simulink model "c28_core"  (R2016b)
settings: Solver=FixedStepDiscrete  StartTime=0.0  StopTime=inf  RelTol=1e-3  EnableMultiTasking=on
undefined symbols (not defined in the file or in its folder): A, ADCIN0, ADCIN1, ADCINA0, ADCINB0, bit, Compare, conversion, DCAEVT1, DCAEVT1FILT, Digital, Down, ended, Event, Filtered, GPTRIP1SEL, GPTRIP2SEL, input, Module, of, Single, start, Trip, TZ1, TZ2, Up, version, Zone
libraries: c2802xlib x36, c280xlib x4, f28M35x_C28x_lib x1, c2000lib x1

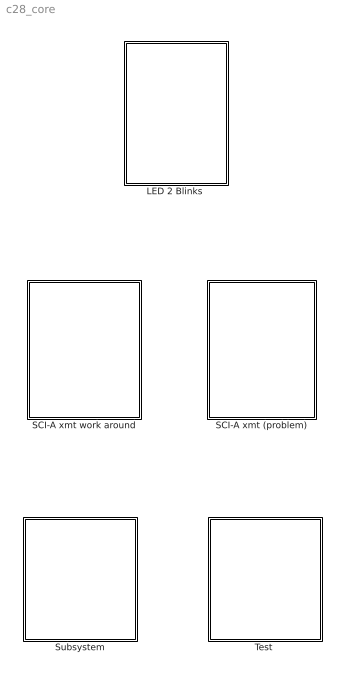
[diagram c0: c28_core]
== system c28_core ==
  "LED 2 Blinks " : Subsystem
  SCI-A xmt (problem) : Subsystem  Commented=on
  SCI-A xmt work around : Subsystem
  Subsystem : Subsystem  Commented=on
  "Test " : Subsystem

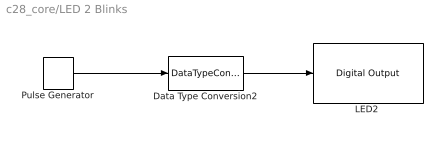
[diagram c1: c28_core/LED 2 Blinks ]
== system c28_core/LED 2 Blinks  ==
  Data Type Conversion2 : DataTypeConversion  OutDataTypeStr=boolean
  "LED2 " : f28M35x_C28x_lib/Digital Output  GPIO_Number=GPIO68~GPIO71  GPIO_Bit0=off  GPIO_BIT0_Toggle=off  GPIO_Bit1=off  GPIO_BIT1_Toggle=off  GPIO_Bit2=off  GPIO_BIT2_Toggle=off  GPIO_Bit3=off  GPIO_BIT3_Toggle=off  GPIO_Bit4=off  GPIO_BIT4_Toggle=off  GPIO_Bit5=off  GPIO_BIT5_Toggle=off  GPIO_Bit6=on  GPIO_BIT6_Toggle=off  GPIO_Bit7=off  GPIO_BIT7_Toggle=off
  Pulse Generator : DiscretePulseGenerator  PulseType=Time based  Period=1  PulseWidth=50
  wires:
  Pulse Generator/1 -> Data Type Conversion2/1
  Data Type Conversion2/1 -> "LED2 "/1

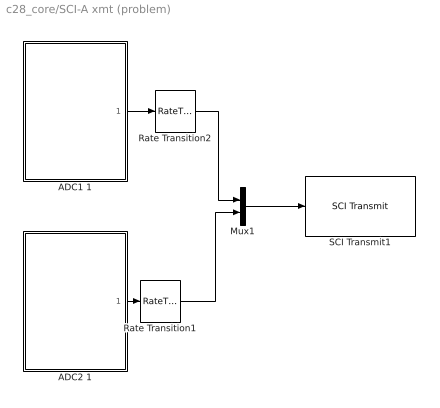
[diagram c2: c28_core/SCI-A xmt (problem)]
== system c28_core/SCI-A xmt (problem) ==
  ADC1 1 : Subsystem
  ADC2 1 : Subsystem
  Mux1 : Mux  Inputs=2
  Rate Transition1 : RateTransition  Deterministic=off
  Rate Transition2 : RateTransition  Deterministic=off
  SCI Transmit1 : c280xlib/SCI Transmit  sciModule=A  dataHead='S'  dataTail='E'  postInterrupt=off  numFifo=1
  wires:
  Mux1/1 -> SCI Transmit1/1
  ADC2 1/1(Out1) -> Rate Transition1/1
  ADC1 1/1(Out1) -> Rate Transition2/1
  Rate Transition2/1 -> Mux1/1
  Rate Transition1/1 -> Mux1/2

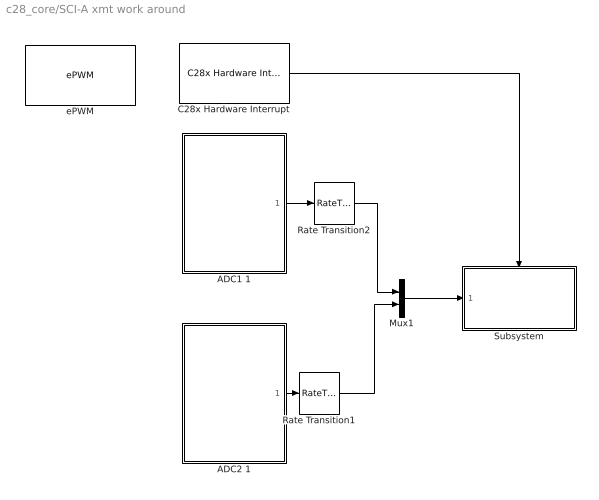
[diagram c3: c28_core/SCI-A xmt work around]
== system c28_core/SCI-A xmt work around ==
  ADC1 1 : Subsystem
  ADC2 1 : Subsystem
  C28x Hardware Interrupt : c2000lib/Scheduling/C28x Hardware Interrupt  irqnumbers=[1]  pienumbers=[1]  irqpriorities=[30]  irqpreempts=[0]  showinput=off  dspchiptype=C280X
  Mux1 : Mux  Inputs=2
  Rate Transition1 : RateTransition  Deterministic=off
  Rate Transition2 : RateTransition  Deterministic=off
  Subsystem : Subsystem
  ePWM : c2802xlib/ePWM  useModule=ePWM6  ePWMxLINKTBPRD=Not Linked  periodUnits=Seconds  timerSource=Specify via dialog  timerPeriod_clk=64000  timerPeriod_sec=0.0001  tbshadow=Counter equals to zero  countingMode=Up-Down  phaseActiveEnable=Disable  phaseDirection=Count down after sync  phaseActive=0  synchronizationEnable=off  dcaevt1Sync=off  dcbevt1Sync=off  synchronizationOption=Disable  clockPrescale=1  HSclockPrescale=1  enswap=off  ePWMxAStatus=on  ePWMxAactionLogic1=Set  ePWMxAactionLogic2=Clear  ePWMxAactionLogic3=Clear  ePWMxAactionLogic4=Set  ePWMxAactionLogic5=Do nothing  ePWMxAactionLogic6=Do nothing  ePWMxALoadMode=Load on counter equals to zero (CTR=Zero)  ePWMxACSFenable=off  ePWMxACSFvalue=Forcing disable  ePWMxASFreload=Zero  ePWMxBStatus=on  ePWMxBactionLogic1=Set  ePWMxBactionLogic2=Clear  ePWMxBactionLogic3=Do nothing  ePWMxBactionLogic4=Do nothing  ePWMxBactionLogic5=Clear  ePWMxBactionLogic6=Set  ePWMxBLoadMode=Load on counter equals to zero (CTR=Zero)  ePWMxBCSFenable=off  ePWMxBCSFvalue=Forcing disable  ePWMxBSFreload=Zero  ePWNxBOutWay=off  ePWMxLINKCMPA=Not Linked  CMPAUnits=Clock cycles  CMPASource=Specify via dialog  CMPAValue_per=50  CMPAValue_clk=32000  enCMPAshadow=Counter equals to zero  ePWMxLINKCMPB=Not Linked  CMPBUnits=Clock cycles  CMPBSource=Specify via dialog  CMPBValue_per=50  CMPBValue_clk=32000  enCMPBshadow=Counter equals to zero  ePWMxLINKCMPC=Not Linked  CMPCUnits=Clock cycles  CMPCSource=Specify via dialog  CMPCValue_per=50  CMPCValue_clk=32000  enCMPCshadow=Counter equals to zero  ePWMxLINKCMPD=Not Linked  CMPDUnits=Clock cycles  CMPDSource=Specify via dialog  CMPDValue_per=50  CMPDValue_clk=32000  enCMPDshadow=Counter equals to zero  enableDBePWMxA=off  enableDBePWMxB=off  enhalfcycle=off  DBpolarity=Active high (AH)  DBedgeDelay=Positive  DBSource_ePWMxA=ePWMxA  DBSource_ePWMxB=ePWMxA  DBperiodSource=Specify via dialog  REDperiod=0  FEDperiod=0  adcstartModuleA=off  adcrequestEventA=First event  adcstartEventA=Digital Compare Module A Event 1 start of conversion (DCAEVT1.soc)  adcstartEventA_type2=Digital Compare Module A Event 1 start of conversion (DCAEVT1.soc)  adcstartModuleB=off  adcrequestEventB=First event  adcstartEventB=Counter equals to zero (CTR=Zero)  adcstartEventB_type2=Counter equals to zero (CTR=Zero)  intEn=on  intPrd=First event  intSel=Counter equals to zero (CTR=Zero)  intSel_type2=Counter equals to zero (CTR=Zero)  hrpe=off  enHRPWM=off  HRPWM_LoadMode=Counter equals to period (CTR=PRD)  HRPWM_CTLMode=Duty or Period control mode  HRPWM_EDGMode=Both edge  hrpeb=off  enHRPWMB=off  HRPWM_LoadModeB=Counter equals to zero (CTR=ZERO)  HRPWM_CTLModeB=Duty or Period control mode  HRPWM_EDGModeB=Both edge  enSFO=on  enautoconv=on  chopperEnable=off  chopperFrequency=1  chopperFirstwidth=1  chopperDuty=12.5%  tripZonesource=Specify via dialog  tzselOSHT1=off  tzselOSHT2=off  tzselOSHT3=off  tzselOSHDCAEV1=off  tzselOSHDCBEV1=off  tzselCBC1=off  tzselCBC2=off  tzselCBC3=off  tzselCBCDCAEV2=off  tzselCBCDCBEV2=off  tzselOSHT4=off  tzselOSHT5=off  tzselOSHT6=off  tzselCBC4=off  tzselCBC5=off  tzselCBC6=off  enTzOstIntr=off  enTzCbcIntr=off  enTzDCAEVT1Intr=off  enTzDCAEVT2Intr=off  enTzDCBEVT1Intr=off  enTzDCBEVT2Intr=off  ePWMxAforced=No action  ePWMxBforced=No action  DCAEVT1forced=No action  DCBEVT1forced=No action  DCAEVT2forced=No action  DCBEVT2forced=No action  dcah=Trip Zone 1 input (TZ1)  dcal=Trip Zone 2 input (TZ2)  dcbh=Trip Zone 1 input (TZ1)  dcbl=Trip Zone 2 input (TZ2)  dcah_type2=GPTRIP1SEL/(TZ1)  dcal_type2=GPTRIP2SEL/(TZ2)  dcbh_type2=GPTRIP1SEL/(TZ1)  dcbl_type2=GPTRIP2SEL/(TZ2)  gendcaevt1=Event disabled  gendcaevt2=Event disabled  gendcbevt1=Event disabled  gendcbevt2=Event disabled  dcaevt1src=DCAEVT1 with sync  dcaevt2src=DCAEVT2 with sync  dcbevt1src=DCBEVT1 with sync  dcbevt2src=DCBEVT2 with sync  pulsesel=Counter equals to zero (CTR=Zero)  blankinv=off  blankoffset=0  blankwidth=0  evsrcsel=Filtered version of DCAEVT1 (DCAEVT1FILT)  encape=off  PwmType=Concerto
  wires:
  Mux1/1 -> Subsystem/1(In1)
  C28x Hardware Interrupt/1 -> Subsystem/Trigger
  ADC2 1/1(Out1) -> Rate Transition1/1
  ADC1 1/1(Out1) -> Rate Transition2/1
  Rate Transition2/1 -> Mux1/1
  Rate Transition1/1 -> Mux1/2

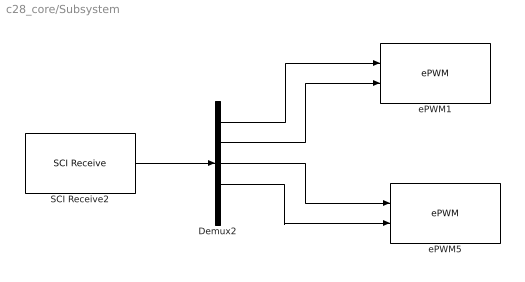
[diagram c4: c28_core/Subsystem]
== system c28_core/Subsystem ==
  Demux2 : Demux  Outputs=5
  SCI Receive2 : c280xlib/SCI Receive  sciModule=A  dataHead='S'  dataTail='E'  dataType=uint16  dataDim=5  initValue=0  errOption=Output the last received value  errValue=0  sampleTime=0.01  outputStatus=off  postInterrupt=off  numFifo=1
  ePWM1 : c2802xlib/ePWM  useModule=ePWM1  ePWMxLINKTBPRD=Not Linked  periodUnits=Clock cycles  timerSource=Specify via dialog  timerPeriod_clk=64000  timerPeriod_sec=0.0001  tbshadow=Counter equals to zero  countingMode=Up-Down  phaseActiveEnable=Disable  phaseDirection=Count down after sync  phaseActive=0  synchronizationEnable=off  dcaevt1Sync=off  dcbevt1Sync=off  synchronizationOption=Disable  clockPrescale=1  HSclockPrescale=1  enswap=off  ePWMxAStatus=on  ePWMxAactionLogic1=Set  ePWMxAactionLogic2=Clear  ePWMxAactionLogic3=Clear  ePWMxAactionLogic4=Set  ePWMxAactionLogic5=Do nothing  ePWMxAactionLogic6=Do nothing  ePWMxALoadMode=Load on counter equals to zero (CTR=Zero)  ePWMxACSFenable=off  ePWMxACSFvalue=Forcing disable  ePWMxASFreload=Zero  ePWMxBStatus=on  ePWMxBactionLogic1=Set  ePWMxBactionLogic2=Clear  ePWMxBactionLogic3=Do nothing  ePWMxBactionLogic4=Do nothing  ePWMxBactionLogic5=Clear  ePWMxBactionLogic6=Set  ePWMxBLoadMode=Load on counter equals to zero (CTR=Zero)  ePWMxBCSFenable=off  ePWMxBCSFvalue=Forcing disable  ePWMxBSFreload=Zero  ePWNxBOutWay=off  ePWMxLINKCMPA=Not Linked  CMPAUnits=Clock cycles  CMPASource=Input port  CMPAValue_per=50  CMPAValue_clk=32000  enCMPAshadow=Counter equals to zero  ePWMxLINKCMPB=Not Linked  CMPBUnits=Clock cycles  CMPBSource=Input port  CMPBValue_per=50  CMPBValue_clk=32000  enCMPBshadow=Counter equals to zero  ePWMxLINKCMPC=Not Linked  CMPCUnits=Clock cycles  CMPCSource=Specify via dialog  CMPCValue_per=50  CMPCValue_clk=32000  enCMPCshadow=Counter equals to zero  ePWMxLINKCMPD=Not Linked  CMPDUnits=Clock cycles  CMPDSource=Specify via dialog  CMPDValue_per=50  CMPDValue_clk=32000  enCMPDshadow=Counter equals to zero  enableDBePWMxA=off  enableDBePWMxB=off  enhalfcycle=off  DBpolarity=Active high (AH)  DBedgeDelay=Positive  DBSource_ePWMxA=ePWMxA  DBSource_ePWMxB=ePWMxA  DBperiodSource=Specify via dialog  REDperiod=0  FEDperiod=0  adcstartModuleA=off  adcrequestEventA=First event  adcstartEventA=Digital Compare Module A Event 1 start of conversion (DCAEVT1.soc)  adcstartEventA_type2=Digital Compare Module A Event 1 start of conversion (DCAEVT1.soc)  adcstartModuleB=off  adcrequestEventB=First event  adcstartEventB=Counter equals to zero (CTR=Zero)  adcstartEventB_type2=Counter equals to zero (CTR=Zero)  intEn=off  intPrd=First event  intSel=Counter equals to zero (CTR=Zero)  intSel_type2=Counter equals to zero (CTR=Zero)  hrpe=off  enHRPWM=off  HRPWM_LoadMode=Counter equals to period (CTR=PRD)  HRPWM_CTLMode=Duty or Period control mode  HRPWM_EDGMode=Both edge  hrpeb=off  enHRPWMB=off  HRPWM_LoadModeB=Counter equals to zero (CTR=ZERO)  HRPWM_CTLModeB=Duty or Period control mode  HRPWM_EDGModeB=Both edge  enSFO=on  enautoconv=on  chopperEnable=off  chopperFrequency=1  chopperFirstwidth=1  chopperDuty=12.5%  tripZonesource=Specify via dialog  tzselOSHT1=off  tzselOSHT2=off  tzselOSHT3=off  tzselOSHDCAEV1=off  tzselOSHDCBEV1=off  tzselCBC1=off  tzselCBC2=off  tzselCBC3=off  tzselCBCDCAEV2=off  tzselCBCDCBEV2=off  tzselOSHT4=off  tzselOSHT5=off  tzselOSHT6=off  tzselCBC4=off  tzselCBC5=off  tzselCBC6=off  enTzOstIntr=off  enTzCbcIntr=off  enTzDCAEVT1Intr=off  enTzDCAEVT2Intr=off  enTzDCBEVT1Intr=off  enTzDCBEVT2Intr=off  ePWMxAforced=No action  ePWMxBforced=No action  DCAEVT1forced=No action  DCBEVT1forced=No action  DCAEVT2forced=No action  DCBEVT2forced=No action  dcah=Trip Zone 1 input (TZ1)  dcal=Trip Zone 2 input (TZ2)  dcbh=Trip Zone 1 input (TZ1)  dcbl=Trip Zone 2 input (TZ2)  dcah_type2=GPTRIP1SEL/(TZ1)  dcal_type2=GPTRIP2SEL/(TZ2)  dcbh_type2=GPTRIP1SEL/(TZ1)  dcbl_type2=GPTRIP2SEL/(TZ2)  gendcaevt1=Event disabled  gendcaevt2=Event disabled  gendcbevt1=Event disabled  gendcbevt2=Event disabled  dcaevt1src=DCAEVT1 with sync  dcaevt2src=DCAEVT2 with sync  dcbevt1src=DCBEVT1 with sync  dcbevt2src=DCBEVT2 with sync  pulsesel=Counter equals to zero (CTR=Zero)  blankinv=off  blankoffset=0  blankwidth=0  evsrcsel=Filtered version of DCAEVT1 (DCAEVT1FILT)  encape=off  PwmType=Concerto
  ePWM5 : c2802xlib/ePWM  useModule=ePWM2  ePWMxLINKTBPRD=Not Linked  periodUnits=Clock cycles  timerSource=Specify via dialog  timerPeriod_clk=64000  timerPeriod_sec=0.0001  tbshadow=Counter equals to zero  countingMode=Up-Down  phaseActiveEnable=Disable  phaseDirection=Count down after sync  phaseActive=0  synchronizationEnable=off  dcaevt1Sync=off  dcbevt1Sync=off  synchronizationOption=Disable  clockPrescale=1  HSclockPrescale=1  enswap=off  ePWMxAStatus=on  ePWMxAactionLogic1=Set  ePWMxAactionLogic2=Clear  ePWMxAactionLogic3=Clear  ePWMxAactionLogic4=Set  ePWMxAactionLogic5=Do nothing  ePWMxAactionLogic6=Do nothing  ePWMxALoadMode=Load on counter equals to zero (CTR=Zero)  ePWMxACSFenable=off  ePWMxACSFvalue=Forcing disable  ePWMxASFreload=Zero  ePWMxBStatus=on  ePWMxBactionLogic1=Set  ePWMxBactionLogic2=Clear  ePWMxBactionLogic3=Do nothing  ePWMxBactionLogic4=Do nothing  ePWMxBactionLogic5=Clear  ePWMxBactionLogic6=Set  ePWMxBLoadMode=Load on counter equals to zero (CTR=Zero)  ePWMxBCSFenable=off  ePWMxBCSFvalue=Forcing disable  ePWMxBSFreload=Zero  ePWNxBOutWay=off  ePWMxLINKCMPA=Not Linked  CMPAUnits=Clock cycles  CMPASource=Input port  CMPAValue_per=50  CMPAValue_clk=32000  enCMPAshadow=Counter equals to zero  ePWMxLINKCMPB=Not Linked  CMPBUnits=Clock cycles  CMPBSource=Input port  CMPBValue_per=50  CMPBValue_clk=32000  enCMPBshadow=Counter equals to zero  ePWMxLINKCMPC=Not Linked  CMPCUnits=Clock cycles  CMPCSource=Specify via dialog  CMPCValue_per=50  CMPCValue_clk=32000  enCMPCshadow=Counter equals to zero  ePWMxLINKCMPD=Not Linked  CMPDUnits=Clock cycles  CMPDSource=Specify via dialog  CMPDValue_per=50  CMPDValue_clk=32000  enCMPDshadow=Counter equals to zero  enableDBePWMxA=off  enableDBePWMxB=off  enhalfcycle=off  DBpolarity=Active high (AH)  DBedgeDelay=Positive  DBSource_ePWMxA=ePWMxA  DBSource_ePWMxB=ePWMxA  DBperiodSource=Specify via dialog  REDperiod=0  FEDperiod=0  adcstartModuleA=off  adcrequestEventA=First event  adcstartEventA=Digital Compare Module A Event 1 start of conversion (DCAEVT1.soc)  adcstartEventA_type2=Digital Compare Module A Event 1 start of conversion (DCAEVT1.soc)  adcstartModuleB=off  adcrequestEventB=First event  adcstartEventB=Counter equals to zero (CTR=Zero)  adcstartEventB_type2=Counter equals to zero (CTR=Zero)  intEn=off  intPrd=First event  intSel=Counter equals to zero (CTR=Zero)  intSel_type2=Counter equals to zero (CTR=Zero)  hrpe=off  enHRPWM=off  HRPWM_LoadMode=Counter equals to period (CTR=PRD)  HRPWM_CTLMode=Duty or Period control mode  HRPWM_EDGMode=Both edge  hrpeb=off  enHRPWMB=off  HRPWM_LoadModeB=Counter equals to zero (CTR=ZERO)  HRPWM_CTLModeB=Duty or Period control mode  HRPWM_EDGModeB=Both edge  enSFO=on  enautoconv=on  chopperEnable=off  chopperFrequency=1  chopperFirstwidth=1  chopperDuty=12.5%  tripZonesource=Specify via dialog  tzselOSHT1=off  tzselOSHT2=off  tzselOSHT3=off  tzselOSHDCAEV1=off  tzselOSHDCBEV1=off  tzselCBC1=off  tzselCBC2=off  tzselCBC3=off  tzselCBCDCAEV2=off  tzselCBCDCBEV2=off  tzselOSHT4=off  tzselOSHT5=off  tzselOSHT6=off  tzselCBC4=off  tzselCBC5=off  tzselCBC6=off  enTzOstIntr=off  enTzCbcIntr=off  enTzDCAEVT1Intr=off  enTzDCAEVT2Intr=off  enTzDCBEVT1Intr=off  enTzDCBEVT2Intr=off  ePWMxAforced=No action  ePWMxBforced=No action  DCAEVT1forced=No action  DCBEVT1forced=No action  DCAEVT2forced=No action  DCBEVT2forced=No action  dcah=Trip Zone 1 input (TZ1)  dcal=Trip Zone 2 input (TZ2)  dcbh=Trip Zone 1 input (TZ1)  dcbl=Trip Zone 2 input (TZ2)  dcah_type2=GPTRIP1SEL/(TZ1)  dcal_type2=GPTRIP2SEL/(TZ2)  dcbh_type2=GPTRIP1SEL/(TZ1)  dcbl_type2=GPTRIP2SEL/(TZ2)  gendcaevt1=Event disabled  gendcaevt2=Event disabled  gendcbevt1=Event disabled  gendcbevt2=Event disabled  dcaevt1src=DCAEVT1 with sync  dcaevt2src=DCAEVT2 with sync  dcbevt1src=DCBEVT1 with sync  dcbevt2src=DCBEVT2 with sync  pulsesel=Counter equals to zero (CTR=Zero)  blankinv=off  blankoffset=0  blankwidth=0  evsrcsel=Filtered version of DCAEVT1 (DCAEVT1FILT)  encape=off  PwmType=Concerto
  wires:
  SCI Receive2/1 -> Demux2/1
  Demux2/4 -> ePWM5/2
  Demux2/3 -> ePWM5/1
  Demux2/2 -> ePWM1/2
  Demux2/1 -> ePWM1/1

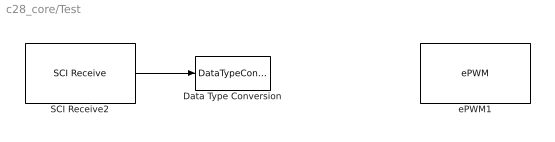
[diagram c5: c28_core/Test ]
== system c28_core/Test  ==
  Data Type Conversion : DataTypeConversion  OutDataTypeStr=uint16
  SCI Receive2 : c280xlib/SCI Receive  sciModule=A  dataHead='S'  dataTail='E'  dataType=uint8  dataDim=1  initValue=0  errOption=Output the last received value  errValue=0  sampleTime=0.01  outputStatus=off  postInterrupt=off  numFifo=1
  ePWM1 : c2802xlib/ePWM  useModule=ePWM1  ePWMxLINKTBPRD=Not Linked  periodUnits=Clock cycles  timerSource=Specify via dialog  timerPeriod_clk=64000  timerPeriod_sec=0.0001  tbshadow=Counter equals to zero  countingMode=Up-Down  phaseActiveEnable=Disable  phaseDirection=Count down after sync  phaseActive=0  synchronizationEnable=off  dcaevt1Sync=off  dcbevt1Sync=off  synchronizationOption=Disable  clockPrescale=1  HSclockPrescale=1  enswap=off  ePWMxAStatus=on  ePWMxAactionLogic1=Set  ePWMxAactionLogic2=Clear  ePWMxAactionLogic3=Clear  ePWMxAactionLogic4=Set  ePWMxAactionLogic5=Do nothing  ePWMxAactionLogic6=Do nothing  ePWMxALoadMode=Load on counter equals to zero (CTR=Zero)  ePWMxACSFenable=off  ePWMxACSFvalue=Forcing disable  ePWMxASFreload=Zero  ePWMxBStatus=on  ePWMxBactionLogic1=Set  ePWMxBactionLogic2=Clear  ePWMxBactionLogic3=Do nothing  ePWMxBactionLogic4=Do nothing  ePWMxBactionLogic5=Clear  ePWMxBactionLogic6=Set  ePWMxBLoadMode=Load on counter equals to zero (CTR=Zero)  ePWMxBCSFenable=off  ePWMxBCSFvalue=Forcing disable  ePWMxBSFreload=Zero  ePWNxBOutWay=off  ePWMxLINKCMPA=Not Linked  CMPAUnits=Clock cycles  CMPASource=Input port  CMPAValue_per=50  CMPAValue_clk=32000  enCMPAshadow=Counter equals to zero  ePWMxLINKCMPB=Not Linked  CMPBUnits=Clock cycles  CMPBSource=Specify via dialog  CMPBValue_per=50  CMPBValue_clk=32000  enCMPBshadow=Counter equals to zero  ePWMxLINKCMPC=Not Linked  CMPCUnits=Clock cycles  CMPCSource=Specify via dialog  CMPCValue_per=50  CMPCValue_clk=32000  enCMPCshadow=Counter equals to zero  ePWMxLINKCMPD=Not Linked  CMPDUnits=Clock cycles  CMPDSource=Specify via dialog  CMPDValue_per=50  CMPDValue_clk=32000  enCMPDshadow=Counter equals to zero  enableDBePWMxA=off  enableDBePWMxB=off  enhalfcycle=off  DBpolarity=Active high (AH)  DBedgeDelay=Positive  DBSource_ePWMxA=ePWMxA  DBSource_ePWMxB=ePWMxA  DBperiodSource=Specify via dialog  REDperiod=0  FEDperiod=0  adcstartModuleA=off  adcrequestEventA=First event  adcstartEventA=Digital Compare Module A Event 1 start of conversion (DCAEVT1.soc)  adcstartEventA_type2=Digital Compare Module A Event 1 start of conversion (DCAEVT1.soc)  adcstartModuleB=off  adcrequestEventB=First event  adcstartEventB=Counter equals to zero (CTR=Zero)  adcstartEventB_type2=Counter equals to zero (CTR=Zero)  intEn=off  intPrd=First event  intSel=Counter equals to zero (CTR=Zero)  intSel_type2=Counter equals to zero (CTR=Zero)  hrpe=off  enHRPWM=off  HRPWM_LoadMode=Counter equals to period (CTR=PRD)  HRPWM_CTLMode=Duty or Period control mode  HRPWM_EDGMode=Both edge  hrpeb=off  enHRPWMB=off  HRPWM_LoadModeB=Counter equals to zero (CTR=ZERO)  HRPWM_CTLModeB=Duty or Period control mode  HRPWM_EDGModeB=Both edge  enSFO=on  enautoconv=on  chopperEnable=off  chopperFrequency=1  chopperFirstwidth=1  chopperDuty=12.5%  tripZonesource=Specify via dialog  tzselOSHT1=off  tzselOSHT2=off  tzselOSHT3=off  tzselOSHDCAEV1=off  tzselOSHDCBEV1=off  tzselCBC1=off  tzselCBC2=off  tzselCBC3=off  tzselCBCDCAEV2=off  tzselCBCDCBEV2=off  tzselOSHT4=off  tzselOSHT5=off  tzselOSHT6=off  tzselCBC4=off  tzselCBC5=off  tzselCBC6=off  enTzOstIntr=off  enTzCbcIntr=off  enTzDCAEVT1Intr=off  enTzDCAEVT2Intr=off  enTzDCBEVT1Intr=off  enTzDCBEVT2Intr=off  ePWMxAforced=No action  ePWMxBforced=No action  DCAEVT1forced=No action  DCBEVT1forced=No action  DCAEVT2forced=No action  DCBEVT2forced=No action  dcah=Trip Zone 1 input (TZ1)  dcal=Trip Zone 2 input (TZ2)  dcbh=Trip Zone 1 input (TZ1)  dcbl=Trip Zone 2 input (TZ2)  dcah_type2=GPTRIP1SEL/(TZ1)  dcal_type2=GPTRIP2SEL/(TZ2)  dcbh_type2=GPTRIP1SEL/(TZ1)  dcbl_type2=GPTRIP2SEL/(TZ2)  gendcaevt1=Event disabled  gendcaevt2=Event disabled  gendcbevt1=Event disabled  gendcbevt2=Event disabled  dcaevt1src=DCAEVT1 with sync  dcaevt2src=DCAEVT2 with sync  dcbevt1src=DCBEVT1 with sync  dcbevt2src=DCBEVT2 with sync  pulsesel=Counter equals to zero (CTR=Zero)  blankinv=off  blankoffset=0  blankwidth=0  evsrcsel=Filtered version of DCAEVT1 (DCAEVT1FILT)  encape=off  PwmType=Concerto
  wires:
  SCI Receive2/1 -> Data Type Conversion/1

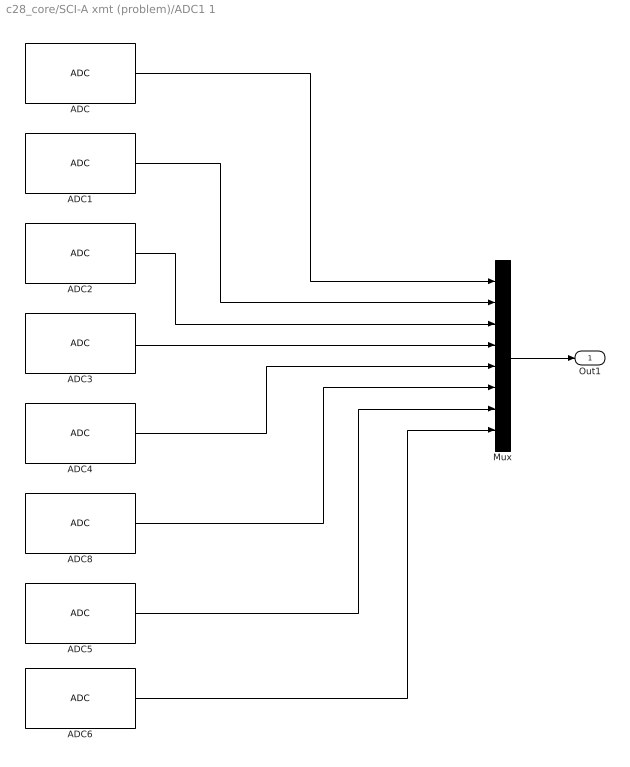
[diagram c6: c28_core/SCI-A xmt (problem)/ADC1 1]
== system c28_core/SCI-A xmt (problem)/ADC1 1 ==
  ADC : c2802xlib/ADC  ADCModule=1  samplingMode=Single sample mode  ADCResolution=12-bit (Single-ended input)  useSOC1=SOC0  useSOC2=SOC0_SOC1  SOCAcquisitionWindow=10  SOCTriggerSource=Software  SOCInterruptTrigger=No ADCINT  Ts=0.0001  dType=uint16  postInterrupt=off  interruptSel=ADCINT1  ADCINTContinuous=off  endma=off  chdma=1  blkParamProc=Concerto  conv1=ADCINA0  conv2=ADCINA0 and ADCINB0  conv1_Type4=ADCIN0  conv2_Type4=ADCIN0 and ADCIN1
  ADC1 : c2802xlib/ADC  ADCModule=1  samplingMode=Single sample mode  ADCResolution=12-bit (Single-ended input)  useSOC1=SOC1  useSOC2=SOC0_SOC1  SOCAcquisitionWindow=10  SOCTriggerSource=Software  SOCInterruptTrigger=No ADCINT  Ts=0.0001  dType=uint16  postInterrupt=off  interruptSel=ADCINT1  ADCINTContinuous=off  endma=off  chdma=1  blkParamProc=Concerto  conv1=ADCINB0  conv2=ADCINA0 and ADCINB0  conv1_Type4=ADCIN0  conv2_Type4=ADCIN0 and ADCIN1
  ADC2 : c2802xlib/ADC  ADCModule=1  samplingMode=Single sample mode  ADCResolution=12-bit (Single-ended input)  useSOC1=SOC2  useSOC2=SOC0_SOC1  SOCAcquisitionWindow=10  SOCTriggerSource=Software  SOCInterruptTrigger=No ADCINT  Ts=0.0001  dType=uint16  postInterrupt=off  interruptSel=ADCINT1  ADCINTContinuous=off  endma=off  chdma=1  blkParamProc=Concerto  conv1=ADCINA2  conv2=ADCINA0 and ADCINB0  conv1_Type4=ADCIN0  conv2_Type4=ADCIN0 and ADCIN1
  ADC3 : c2802xlib/ADC  ADCModule=1  samplingMode=Single sample mode  ADCResolution=12-bit (Single-ended input)  useSOC1=SOC3  useSOC2=SOC0_SOC1  SOCAcquisitionWindow=10  SOCTriggerSource=Software  SOCInterruptTrigger=No ADCINT  Ts=0.0001  dType=uint16  postInterrupt=off  interruptSel=ADCINT1  ADCINTContinuous=off  endma=off  chdma=1  blkParamProc=Concerto  conv1=ADCINA3  conv2=ADCINA0 and ADCINB0  conv1_Type4=ADCIN0  conv2_Type4=ADCIN0 and ADCIN1
  ADC4 : c2802xlib/ADC  ADCModule=1  samplingMode=Single sample mode  ADCResolution=12-bit (Single-ended input)  useSOC1=SOC4  useSOC2=SOC0_SOC1  SOCAcquisitionWindow=10  SOCTriggerSource=Software  SOCInterruptTrigger=No ADCINT  Ts=0.0001  dType=uint16  postInterrupt=off  interruptSel=ADCINT1  ADCINTContinuous=off  endma=off  chdma=1  blkParamProc=Concerto  conv1=ADCINA4  conv2=ADCINA0 and ADCINB0  conv1_Type4=ADCIN0  conv2_Type4=ADCIN0 and ADCIN1
  ADC5 : c2802xlib/ADC  ADCModule=1  samplingMode=Single sample mode  ADCResolution=12-bit (Single-ended input)  useSOC1=SOC6  useSOC2=SOC0_SOC1  SOCAcquisitionWindow=10  SOCTriggerSource=Software  SOCInterruptTrigger=No ADCINT  Ts=0.0001  dType=uint16  postInterrupt=off  interruptSel=ADCINT1  ADCINTContinuous=off  endma=off  chdma=1  blkParamProc=Concerto  conv1=ADCINA6  conv2=ADCINA0 and ADCINB0  conv1_Type4=ADCIN0  conv2_Type4=ADCIN0 and ADCIN1
  ADC6 : c2802xlib/ADC  ADCModule=1  samplingMode=Single sample mode  ADCResolution=12-bit (Single-ended input)  useSOC1=SOC7  useSOC2=SOC0_SOC1  SOCAcquisitionWindow=10  SOCTriggerSource=Software  SOCInterruptTrigger=No ADCINT  Ts=0.0001  dType=uint16  postInterrupt=on  interruptSel=ADCINT1  ADCINTContinuous=off  endma=off  chdma=1  blkParamProc=Concerto  conv1=ADCINA7  conv2=ADCINA0 and ADCINB0  conv1_Type4=ADCIN0  conv2_Type4=ADCIN0 and ADCIN1
  ADC8 : c2802xlib/ADC  ADCModule=1  samplingMode=Single sample mode  ADCResolution=12-bit (Single-ended input)  useSOC1=SOC5  useSOC2=SOC0_SOC1  SOCAcquisitionWindow=10  SOCTriggerSource=Software  SOCInterruptTrigger=No ADCINT  Ts=0.0001  dType=uint16  postInterrupt=off  interruptSel=ADCINT1  ADCINTContinuous=off  endma=off  chdma=1  blkParamProc=Concerto  conv1=ADCINB4  conv2=ADCINA0 and ADCINB0  conv1_Type4=ADCIN0  conv2_Type4=ADCIN0 and ADCIN1
  Mux : Mux  Inputs=8
  Out1 : Outport
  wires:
  Mux/1 -> Out1/1
  ADC/1 -> Mux/1
  ADC1/1 -> Mux/2
  ADC2/1 -> Mux/3
  ADC3/1 -> Mux/4
  ADC4/1 -> Mux/5
  ADC8/1 -> Mux/6
  ADC5/1 -> Mux/7
  ADC6/1 -> Mux/8

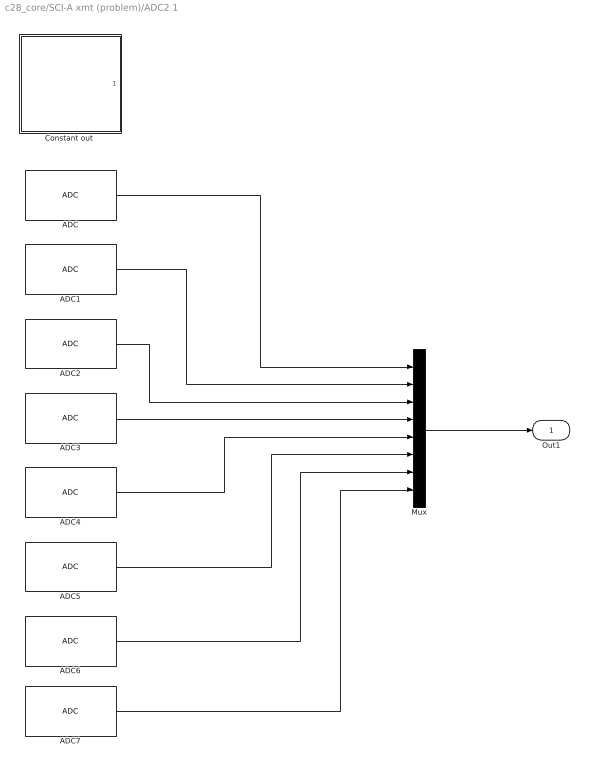
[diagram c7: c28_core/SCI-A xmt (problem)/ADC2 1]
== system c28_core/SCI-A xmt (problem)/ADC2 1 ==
  ADC : c2802xlib/ADC  ADCModule=2  samplingMode=Single sample mode  ADCResolution=12-bit (Single-ended input)  useSOC1=SOC8  useSOC2=SOC0_SOC1  SOCAcquisitionWindow=10  SOCTriggerSource=Software  SOCInterruptTrigger=No ADCINT  Ts=0.0001  dType=uint16  postInterrupt=off  interruptSel=ADCINT1  ADCINTContinuous=off  endma=off  chdma=1  blkParamProc=Concerto  conv1=ADCINA0  conv2=ADCINA0 and ADCINB0  conv1_Type4=ADCIN0  conv2_Type4=ADCIN0 and ADCIN1
  ADC1 : c2802xlib/ADC  ADCModule=2  samplingMode=Single sample mode  ADCResolution=12-bit (Single-ended input)  useSOC1=SOC9  useSOC2=SOC0_SOC1  SOCAcquisitionWindow=10  SOCTriggerSource=Software  SOCInterruptTrigger=No ADCINT  Ts=0.0001  dType=uint16  postInterrupt=off  interruptSel=ADCINT1  ADCINTContinuous=off  endma=off  chdma=1  blkParamProc=Concerto  conv1=ADCINB0  conv2=ADCINA0 and ADCINB0  conv1_Type4=ADCIN0  conv2_Type4=ADCIN0 and ADCIN1
  ADC2 : c2802xlib/ADC  ADCModule=2  samplingMode=Single sample mode  ADCResolution=12-bit (Single-ended input)  useSOC1=SOC10  useSOC2=SOC0_SOC1  SOCAcquisitionWindow=10  SOCTriggerSource=Software  SOCInterruptTrigger=No ADCINT  Ts=0.0001  dType=uint16  postInterrupt=off  interruptSel=ADCINT1  ADCINTContinuous=off  endma=off  chdma=1  blkParamProc=Concerto  conv1=ADCINA2  conv2=ADCINA0 and ADCINB0  conv1_Type4=ADCIN0  conv2_Type4=ADCIN0 and ADCIN1
  ADC3 : c2802xlib/ADC  ADCModule=2  samplingMode=Single sample mode  ADCResolution=12-bit (Single-ended input)  useSOC1=SOC11  useSOC2=SOC0_SOC1  SOCAcquisitionWindow=10  SOCTriggerSource=Software  SOCInterruptTrigger=No ADCINT  Ts=0.0001  dType=uint16  postInterrupt=off  interruptSel=ADCINT1  ADCINTContinuous=off  endma=off  chdma=1  blkParamProc=Concerto  conv1=ADCINA3  conv2=ADCINA0 and ADCINB0  conv1_Type4=ADCIN0  conv2_Type4=ADCIN0 and ADCIN1
  ADC4 : c2802xlib/ADC  ADCModule=2  samplingMode=Single sample mode  ADCResolution=12-bit (Single-ended input)  useSOC1=SOC12  useSOC2=SOC0_SOC1  SOCAcquisitionWindow=10  SOCTriggerSource=Software  SOCInterruptTrigger=No ADCINT  Ts=0.0001  dType=uint16  postInterrupt=off  interruptSel=ADCINT1  ADCINTContinuous=off  endma=off  chdma=1  blkParamProc=Concerto  conv1=ADCINA4  conv2=ADCINA0 and ADCINB0  conv1_Type4=ADCIN0  conv2_Type4=ADCIN0 and ADCIN1
  ADC5 : c2802xlib/ADC  ADCModule=2  samplingMode=Single sample mode  ADCResolution=12-bit (Single-ended input)  useSOC1=SOC13  useSOC2=SOC0_SOC1  SOCAcquisitionWindow=10  SOCTriggerSource=Software  SOCInterruptTrigger=No ADCINT  Ts=0.0001  dType=uint16  postInterrupt=off  interruptSel=ADCINT1  ADCINTContinuous=off  endma=off  chdma=1  blkParamProc=Concerto  conv1=ADCINB4  conv2=ADCINA0 and ADCINB0  conv1_Type4=ADCIN0  conv2_Type4=ADCIN0 and ADCIN1
  ADC6 : c2802xlib/ADC  ADCModule=2  samplingMode=Single sample mode  ADCResolution=12-bit (Single-ended input)  useSOC1=SOC14  useSOC2=SOC0_SOC1  SOCAcquisitionWindow=10  SOCTriggerSource=Software  SOCInterruptTrigger=No ADCINT  Ts=0.0001  dType=uint16  postInterrupt=off  interruptSel=ADCINT1  ADCINTContinuous=off  endma=off  chdma=1  blkParamProc=Concerto  conv1=ADCINA6  conv2=ADCINA0 and ADCINB0  conv1_Type4=ADCIN0  conv2_Type4=ADCIN0 and ADCIN1
  ADC7 : c2802xlib/ADC  ADCModule=2  samplingMode=Single sample mode  ADCResolution=12-bit (Single-ended input)  useSOC1=SOC15  useSOC2=SOC0_SOC1  SOCAcquisitionWindow=10  SOCTriggerSource=Software  SOCInterruptTrigger=No ADCINT  Ts=0.0001  dType=uint16  postInterrupt=off  interruptSel=ADCINT1  ADCINTContinuous=off  endma=off  chdma=1  blkParamProc=Concerto  conv1=ADCINA7  conv2=ADCINA0 and ADCINB0  conv1_Type4=ADCIN0  conv2_Type4=ADCIN0 and ADCIN1
  "Constant out " : Subsystem  Commented=on
  Mux : Mux  Inputs=8
  Out1 : Outport
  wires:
  ADC/1 -> Mux/1
  ADC1/1 -> Mux/2
  ADC2/1 -> Mux/3
  ADC3/1 -> Mux/4
  ADC4/1 -> Mux/5
  ADC5/1 -> Mux/6
  ADC6/1 -> Mux/7
  ADC7/1 -> Mux/8
  Mux/1 -> Out1/1

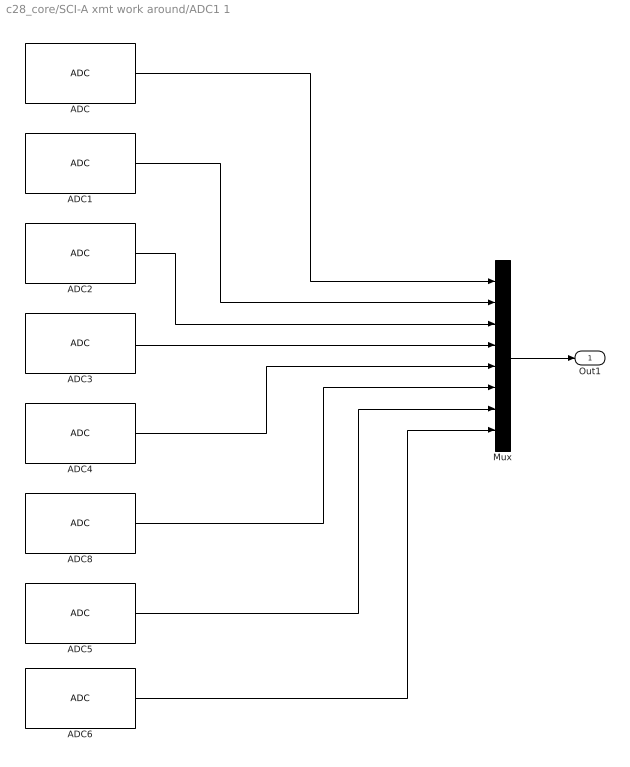
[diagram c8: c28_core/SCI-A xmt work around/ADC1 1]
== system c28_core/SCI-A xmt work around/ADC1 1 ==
  ADC : c2802xlib/ADC  ADCModule=1  samplingMode=Single sample mode  ADCResolution=12-bit (Single-ended input)  useSOC1=SOC0  useSOC2=SOC0_SOC1  SOCAcquisitionWindow=10  SOCTriggerSource=Software  SOCInterruptTrigger=No ADCINT  Ts=0.0001  dType=uint16  postInterrupt=off  interruptSel=ADCINT1  ADCINTContinuous=off  endma=off  chdma=1  blkParamProc=Concerto  conv1=ADCINA0  conv2=ADCINA0 and ADCINB0  conv1_Type4=ADCIN0  conv2_Type4=ADCIN0 and ADCIN1
  ADC1 : c2802xlib/ADC  ADCModule=1  samplingMode=Single sample mode  ADCResolution=12-bit (Single-ended input)  useSOC1=SOC1  useSOC2=SOC0_SOC1  SOCAcquisitionWindow=10  SOCTriggerSource=Software  SOCInterruptTrigger=No ADCINT  Ts=0.0001  dType=uint16  postInterrupt=off  interruptSel=ADCINT1  ADCINTContinuous=off  endma=off  chdma=1  blkParamProc=Concerto  conv1=ADCINB0  conv2=ADCINA0 and ADCINB0  conv1_Type4=ADCIN0  conv2_Type4=ADCIN0 and ADCIN1
  ADC2 : c2802xlib/ADC  ADCModule=1  samplingMode=Single sample mode  ADCResolution=12-bit (Single-ended input)  useSOC1=SOC2  useSOC2=SOC0_SOC1  SOCAcquisitionWindow=10  SOCTriggerSource=Software  SOCInterruptTrigger=No ADCINT  Ts=0.0001  dType=uint16  postInterrupt=off  interruptSel=ADCINT1  ADCINTContinuous=off  endma=off  chdma=1  blkParamProc=Concerto  conv1=ADCINA2  conv2=ADCINA0 and ADCINB0  conv1_Type4=ADCIN0  conv2_Type4=ADCIN0 and ADCIN1
  ADC3 : c2802xlib/ADC  ADCModule=1  samplingMode=Single sample mode  ADCResolution=12-bit (Single-ended input)  useSOC1=SOC3  useSOC2=SOC0_SOC1  SOCAcquisitionWindow=10  SOCTriggerSource=Software  SOCInterruptTrigger=No ADCINT  Ts=0.0001  dType=uint16  postInterrupt=off  interruptSel=ADCINT1  ADCINTContinuous=off  endma=off  chdma=1  blkParamProc=Concerto  conv1=ADCINA3  conv2=ADCINA0 and ADCINB0  conv1_Type4=ADCIN0  conv2_Type4=ADCIN0 and ADCIN1
  ADC4 : c2802xlib/ADC  ADCModule=1  samplingMode=Single sample mode  ADCResolution=12-bit (Single-ended input)  useSOC1=SOC4  useSOC2=SOC0_SOC1  SOCAcquisitionWindow=10  SOCTriggerSource=Software  SOCInterruptTrigger=No ADCINT  Ts=0.0001  dType=uint16  postInterrupt=off  interruptSel=ADCINT1  ADCINTContinuous=off  endma=off  chdma=1  blkParamProc=Concerto  conv1=ADCINA4  conv2=ADCINA0 and ADCINB0  conv1_Type4=ADCIN0  conv2_Type4=ADCIN0 and ADCIN1
  ADC5 : c2802xlib/ADC  ADCModule=1  samplingMode=Single sample mode  ADCResolution=12-bit (Single-ended input)  useSOC1=SOC6  useSOC2=SOC0_SOC1  SOCAcquisitionWindow=10  SOCTriggerSource=Software  SOCInterruptTrigger=No ADCINT  Ts=0.0001  dType=uint16  postInterrupt=off  interruptSel=ADCINT1  ADCINTContinuous=off  endma=off  chdma=1  blkParamProc=Concerto  conv1=ADCINA6  conv2=ADCINA0 and ADCINB0  conv1_Type4=ADCIN0  conv2_Type4=ADCIN0 and ADCIN1
  ADC6 : c2802xlib/ADC  ADCModule=1  samplingMode=Single sample mode  ADCResolution=12-bit (Single-ended input)  useSOC1=SOC7  useSOC2=SOC0_SOC1  SOCAcquisitionWindow=10  SOCTriggerSource=Software  SOCInterruptTrigger=No ADCINT  Ts=0.0001  dType=uint16  postInterrupt=on  interruptSel=ADCINT1  ADCINTContinuous=off  endma=off  chdma=1  blkParamProc=Concerto  conv1=ADCINA7  conv2=ADCINA0 and ADCINB0  conv1_Type4=ADCIN0  conv2_Type4=ADCIN0 and ADCIN1
  ADC8 : c2802xlib/ADC  ADCModule=1  samplingMode=Single sample mode  ADCResolution=12-bit (Single-ended input)  useSOC1=SOC5  useSOC2=SOC0_SOC1  SOCAcquisitionWindow=10  SOCTriggerSource=Software  SOCInterruptTrigger=No ADCINT  Ts=0.0001  dType=uint16  postInterrupt=off  interruptSel=ADCINT1  ADCINTContinuous=off  endma=off  chdma=1  blkParamProc=Concerto  conv1=ADCINB4  conv2=ADCINA0 and ADCINB0  conv1_Type4=ADCIN0  conv2_Type4=ADCIN0 and ADCIN1
  Mux : Mux  Inputs=8
  Out1 : Outport
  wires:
  Mux/1 -> Out1/1
  ADC/1 -> Mux/1
  ADC1/1 -> Mux/2
  ADC2/1 -> Mux/3
  ADC3/1 -> Mux/4
  ADC4/1 -> Mux/5
  ADC8/1 -> Mux/6
  ADC5/1 -> Mux/7
  ADC6/1 -> Mux/8

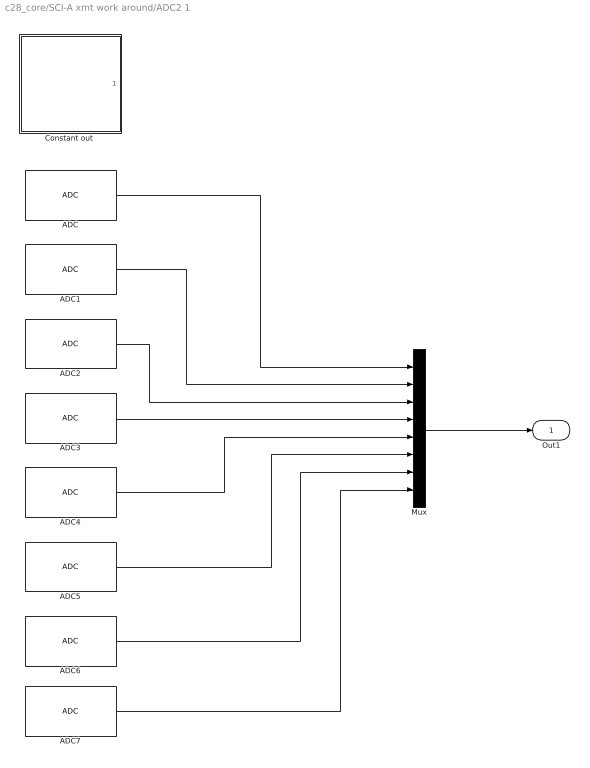
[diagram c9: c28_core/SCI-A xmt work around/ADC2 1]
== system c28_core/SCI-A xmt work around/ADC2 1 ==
  ADC : c2802xlib/ADC  ADCModule=2  samplingMode=Single sample mode  ADCResolution=12-bit (Single-ended input)  useSOC1=SOC8  useSOC2=SOC0_SOC1  SOCAcquisitionWindow=10  SOCTriggerSource=Software  SOCInterruptTrigger=No ADCINT  Ts=0.0001  dType=uint16  postInterrupt=off  interruptSel=ADCINT1  ADCINTContinuous=off  endma=off  chdma=1  blkParamProc=Concerto  conv1=ADCINA0  conv2=ADCINA0 and ADCINB0  conv1_Type4=ADCIN0  conv2_Type4=ADCIN0 and ADCIN1
  ADC1 : c2802xlib/ADC  ADCModule=2  samplingMode=Single sample mode  ADCResolution=12-bit (Single-ended input)  useSOC1=SOC9  useSOC2=SOC0_SOC1  SOCAcquisitionWindow=10  SOCTriggerSource=Software  SOCInterruptTrigger=No ADCINT  Ts=0.0001  dType=uint16  postInterrupt=off  interruptSel=ADCINT1  ADCINTContinuous=off  endma=off  chdma=1  blkParamProc=Concerto  conv1=ADCINB0  conv2=ADCINA0 and ADCINB0  conv1_Type4=ADCIN0  conv2_Type4=ADCIN0 and ADCIN1
  ADC2 : c2802xlib/ADC  ADCModule=2  samplingMode=Single sample mode  ADCResolution=12-bit (Single-ended input)  useSOC1=SOC10  useSOC2=SOC0_SOC1  SOCAcquisitionWindow=10  SOCTriggerSource=Software  SOCInterruptTrigger=No ADCINT  Ts=0.0001  dType=uint16  postInterrupt=off  interruptSel=ADCINT1  ADCINTContinuous=off  endma=off  chdma=1  blkParamProc=Concerto  conv1=ADCINA2  conv2=ADCINA0 and ADCINB0  conv1_Type4=ADCIN0  conv2_Type4=ADCIN0 and ADCIN1
  ADC3 : c2802xlib/ADC  ADCModule=2  samplingMode=Single sample mode  ADCResolution=12-bit (Single-ended input)  useSOC1=SOC11  useSOC2=SOC0_SOC1  SOCAcquisitionWindow=10  SOCTriggerSource=Software  SOCInterruptTrigger=No ADCINT  Ts=0.0001  dType=uint16  postInterrupt=off  interruptSel=ADCINT1  ADCINTContinuous=off  endma=off  chdma=1  blkParamProc=Concerto  conv1=ADCINA3  conv2=ADCINA0 and ADCINB0  conv1_Type4=ADCIN0  conv2_Type4=ADCIN0 and ADCIN1
  ADC4 : c2802xlib/ADC  ADCModule=2  samplingMode=Single sample mode  ADCResolution=12-bit (Single-ended input)  useSOC1=SOC12  useSOC2=SOC0_SOC1  SOCAcquisitionWindow=10  SOCTriggerSource=Software  SOCInterruptTrigger=No ADCINT  Ts=0.0001  dType=uint16  postInterrupt=off  interruptSel=ADCINT1  ADCINTContinuous=off  endma=off  chdma=1  blkParamProc=Concerto  conv1=ADCINA4  conv2=ADCINA0 and ADCINB0  conv1_Type4=ADCIN0  conv2_Type4=ADCIN0 and ADCIN1
  ADC5 : c2802xlib/ADC  ADCModule=2  samplingMode=Single sample mode  ADCResolution=12-bit (Single-ended input)  useSOC1=SOC13  useSOC2=SOC0_SOC1  SOCAcquisitionWindow=10  SOCTriggerSource=Software  SOCInterruptTrigger=No ADCINT  Ts=0.0001  dType=uint16  postInterrupt=off  interruptSel=ADCINT1  ADCINTContinuous=off  endma=off  chdma=1  blkParamProc=Concerto  conv1=ADCINB4  conv2=ADCINA0 and ADCINB0  conv1_Type4=ADCIN0  conv2_Type4=ADCIN0 and ADCIN1
  ADC6 : c2802xlib/ADC  ADCModule=2  samplingMode=Single sample mode  ADCResolution=12-bit (Single-ended input)  useSOC1=SOC14  useSOC2=SOC0_SOC1  SOCAcquisitionWindow=10  SOCTriggerSource=Software  SOCInterruptTrigger=No ADCINT  Ts=0.0001  dType=uint16  postInterrupt=off  interruptSel=ADCINT1  ADCINTContinuous=off  endma=off  chdma=1  blkParamProc=Concerto  conv1=ADCINA6  conv2=ADCINA0 and ADCINB0  conv1_Type4=ADCIN0  conv2_Type4=ADCIN0 and ADCIN1
  ADC7 : c2802xlib/ADC  ADCModule=2  samplingMode=Single sample mode  ADCResolution=12-bit (Single-ended input)  useSOC1=SOC15  useSOC2=SOC0_SOC1  SOCAcquisitionWindow=10  SOCTriggerSource=Software  SOCInterruptTrigger=No ADCINT  Ts=0.0001  dType=uint16  postInterrupt=off  interruptSel=ADCINT1  ADCINTContinuous=off  endma=off  chdma=1  blkParamProc=Concerto  conv1=ADCINA7  conv2=ADCINA0 and ADCINB0  conv1_Type4=ADCIN0  conv2_Type4=ADCIN0 and ADCIN1
  "Constant out " : Subsystem  Commented=on
  Mux : Mux  Inputs=8
  Out1 : Outport
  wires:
  ADC/1 -> Mux/1
  ADC1/1 -> Mux/2
  ADC2/1 -> Mux/3
  ADC3/1 -> Mux/4
  ADC4/1 -> Mux/5
  ADC5/1 -> Mux/6
  ADC6/1 -> Mux/7
  ADC7/1 -> Mux/8
  Mux/1 -> Out1/1

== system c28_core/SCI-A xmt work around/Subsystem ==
  In1 : Inport
  function : TriggerPort  TriggerType=function-call  VariantControl=Variant
  SCI Transmit1 : c280xlib/SCI Transmit  sciModule=A  dataHead='S'  dataTail='E'  postInterrupt=off  numFifo=1
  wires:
  In1/1 -> SCI Transmit1/1

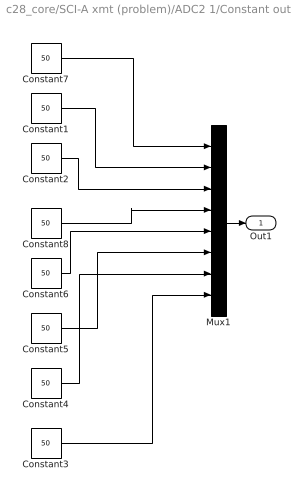
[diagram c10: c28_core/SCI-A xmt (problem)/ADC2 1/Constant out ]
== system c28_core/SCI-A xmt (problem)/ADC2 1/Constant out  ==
  Constant{1..8} (8 alike) : Constant  Commented=on  Value=50  OutDataTypeStr=uint16
  Mux1 : Mux  Commented=on  Inputs=8
  Out1 : Outport
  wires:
  Mux1/1 -> Out1/1
  Constant7/1 -> Mux1/1
  Constant5/1 -> Mux1/6
  Constant8/1 -> Mux1/4
  Constant3/1 -> Mux1/8
  Constant1/1 -> Mux1/2
  Constant6/1 -> Mux1/5
  Constant2/1 -> Mux1/3
  Constant4/1 -> Mux1/7

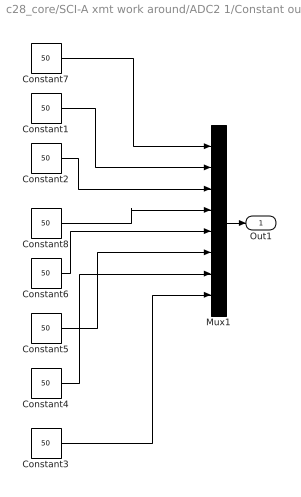
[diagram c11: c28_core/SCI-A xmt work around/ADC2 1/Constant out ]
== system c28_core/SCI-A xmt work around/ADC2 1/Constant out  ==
  Constant{1..8} (8 alike) : Constant  Commented=on  Value=50  OutDataTypeStr=uint16
  Mux1 : Mux  Commented=on  Inputs=8
  Out1 : Outport
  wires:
  Mux1/1 -> Out1/1
  Constant7/1 -> Mux1/1
  Constant5/1 -> Mux1/6
  Constant8/1 -> Mux1/4
  Constant3/1 -> Mux1/8
  Constant1/1 -> Mux1/2
  Constant6/1 -> Mux1/5
  Constant2/1 -> Mux1/3
  Constant4/1 -> Mux1/7
